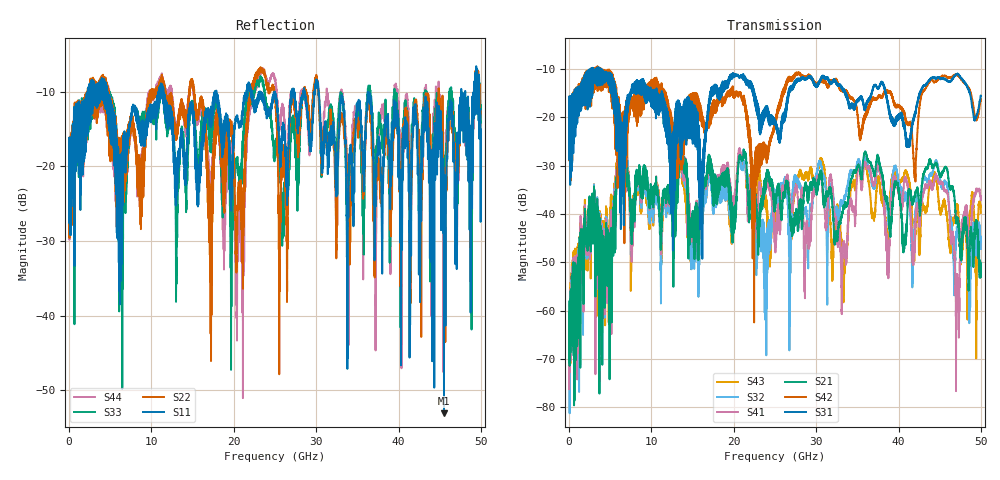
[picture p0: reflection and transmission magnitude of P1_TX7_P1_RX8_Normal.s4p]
!Keysight Technologies,N5225B,MY57041031,A.13.20.10
!Date: Friday, May 31, 2019 11:26:15
!Correction: S11(Full 4 Port(1,2,3,4))
!S12(Full 4 Port(1,2,3,4))
!S13(Full 4 Port(1,2,3,4))
!S14(Full 4 Port(1,2,3,4))
!S21(Full 4 Port(1,2,3,4))
!S22(Full 4 Port(1,2,3,4))
!S23(Full 4 Port(1,2,3,4))
!S24(Full 4 Port(1,2,3,4))
!S31(Full 4 Port(1,2,3,4))
!S32(Full 4 Port(1,2,3,4))
!S33(Full 4 Port(1,2,3,4))
!S34(Full 4 Port(1,2,3,4))
!S41(Full 4 Port(1,2,3,4))
!S42(Full 4 Port(1,2,3,4))
!S43(Full 4 Port(1,2,3,4))
!S44(Full 4 Port(1,2,3,4))
!S4P File: Measurements: <S11,S12,S13,S14>,
!<S21,S22,S23,S24>,
!<S31,S32,S33,S34>,
!<S41,S42,S43,S44>:
# Hz S  dB  R 50.0
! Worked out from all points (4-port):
!   5000 points, 10 MHz to 50 GHz, reference 50 ohm
!   strongest paths, dB at 10 MHz, 12.51 GHz, 25.01 GHz, 37.51 GHz, 50 GHz:
!     S31: -19.3, -39.4, -20.9, -14.0, -15.5
!     S42: -19.3, -24.2, -21.8, -15.8, -16.3
!     S21: -58.1, -38.8, -38.2, -28.0, -52.7
!     S41: -61.6, -34.8, -46.8, -30.3, -36.7
!     S32: -63.8, -36.6, -36.9, -29.5, -47.3
!     S43: -63.0, -32.9, -42.0, -32.6, -39.8
!   lowest |S11| = -53.1 dB at 45.52 GHz (marker M1), VSWR 1.00, Z = 49.8 + j0.15 ohm
!   |S11| at or under -10 dB: 4.613 GHz to 10.86 GHz (6.247 GHz wide, 80.8 % of centre); 11.46 GHz to 17.74 GHz (6.282 GHz wide, 43 % of centre); 30.28 GHz to 47.6 GHz (17.32 GHz wide, 44.5 % of centre)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
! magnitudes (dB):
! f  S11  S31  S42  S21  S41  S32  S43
! 10 MHz  -19.4  -19.3  -19.3  -58.1  -61.6  -63.8  -63.0
! 6.22 GHz  -26.7  -19.9  -20.1  -28.0  -27.5  -27.2  -26.3
! 20.38 GHz  -13.4  -11.2  -14.7  -35.2  -32.6  -34.5  -32.8
! 23.9 GHz  -13.0  -19.3  -28.7  -34.4  -34.9  -57.7  -39.0
! 45.52 GHz  -53.1  -12.0  -11.5  -30.7  -34.8  -34.1  -37.2
! 47.15 GHz  -16.0  -10.9  -11.3  -41.5  -53.9  -43.6  -38.4
! 50 GHz  -15.1  -15.5  -16.3  -52.7  -36.7  -47.3  -39.8
